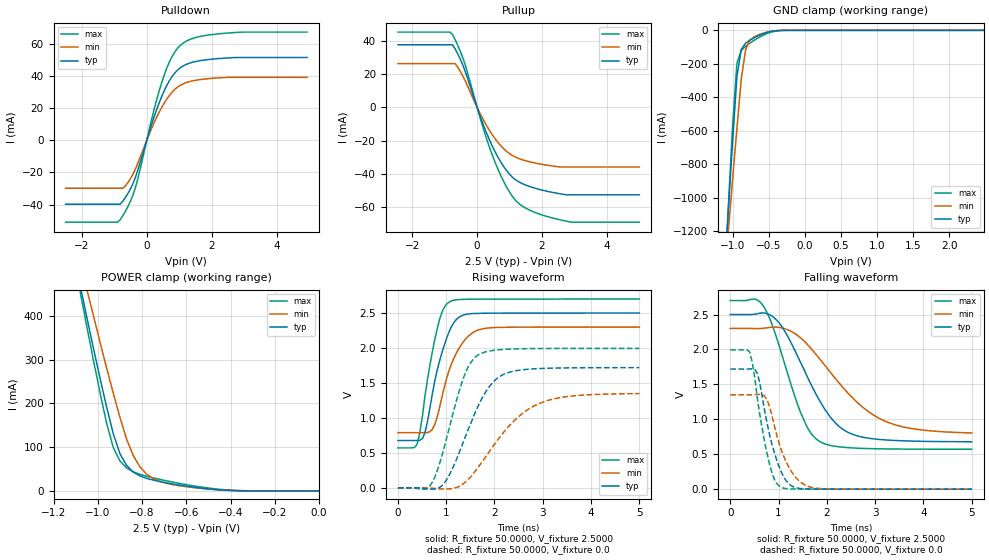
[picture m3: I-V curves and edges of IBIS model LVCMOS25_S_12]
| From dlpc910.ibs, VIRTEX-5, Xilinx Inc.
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|   Model LVCMOS25_S_12
[Model]  LVCMOS25_S_12
Model_type I/O
Polarity   Non-Inverting
Enable   Active-Low
Vinl = 0.65
Vinh = 1.85
Vmeas =  1.2500V
Cref =   0.0F
Rref =   1.0000M
Vref =   0.0V
C_comp   6.0000pF   6.0000pF   6.0000pF
[Model Spec]
Vinl   0.65   0.6   0.7
Vinh   1.85   1.7   2.0
[Temperature Range]   25.0000   85.0000   0.0
[Voltage Range]   2.5000V   2.3000V   2.7000V
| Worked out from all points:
|   slope of the pulldown table from 0 to 0.375 V, typ, clamps not added: 16.3 ohm
|   slope of the pullup table from 0 to 0.375 V, typ, clamps not added: 19.5 ohm
|   GND clamp passes 1 mA (typ) near -0.35 V on its own axis
|   POWER clamp passes 1 mA (typ) near -0.40 V on its own axis
|   rising waveform, R_fixture 50.0000, V_fixture 2.5000: 20-80 % time 370ps typ, 426ps min, 312ps max; typ from 0.677 V to 2.5 V
|   rising waveform, R_fixture 50.0000, V_fixture 0.0: 20-80 % time 648ps typ, 971ps min, 486ps max; typ from 0 V to 1.72 V
|   falling waveform, R_fixture 50.0000, V_fixture 2.5000: 20-80 % time 831ps typ, 1.19ns min, 613ps max; typ from 2.5 V to 0.679 V
|   falling waveform, R_fixture 50.0000, V_fixture 0.0: 20-80 % time 350ps typ, 399ps min, 293ps max; typ from 1.72 V to 0 V
[Pulldown]
|Voltage   I(typ)   I(min)   I(max)
-2.5V     -39.8mA    -29.84mA   -51mA
-900mV    -39.8mA    -29.84mA   -51mA
-820mV    -39.8mA    -29.84mA   -49.53mA
-660mV    -35.7mA    -28.49mA   -44.35mA
-340mV    -22.55mA   -17.45mA   -28.94mA
220mV     14.2mA     10.7mA     18.76mA
540mV     30.98mA    23.3mA     40.82mA
780mV     39.81mA    30.03mA    52.29mA
1.1V      46.18mA    35.06mA    60.36mA
1.5V      49.17mA    37.49mA    64.12mA
2.22V     51.04mA    39.01mA    66.47mA
4.94V     51.73mA    39.36mA    67.56mA
[Pullup]
|Voltage   I(typ)   I(min)   I(max)
-2.44V    37.46mA    26.15mA    45.04mA
-840mV    37.46mA    26.15mA    45.04mA
-760mV    37.46mA    26.15mA    43.62mA
-600mV    32.11mA    24.14mA    37.29mA
-360mV    21.09mA    15.58mA    24.96mA
120mV     -6.701mA   -4.795mA   -8.164mA
520mV     -25.32mA   -17.91mA   -31.29mA
920mV     -38.23mA   -26.59mA   -48.16mA
1.32V     -45.02mA   -30.95mA   -58.15mA
1.96V     -49.41mA   -34.03mA   -64.25mA
2.92V     -52.44mA   -35.78mA   -68.84mA
5V        -52.44mA   -35.78mA   -68.84mA
[GND_clamp]
|Voltage   I(typ)   I(min)   I(max)
-2.5V     -11.29A    -8.704A    -13.53A
-1.12V    -1.497A    -1.51A     -1.57A
-1.06V    -1.075A    -1.198A    -1.059A
-1V       -662mA     -888.5mA   -563.2mA
-940mV    -273.6mA   -582.9mA   -195.1mA
-880mV    -113.7mA   -290.3mA   -119.7mA
-820mV    -76.4mA    -115.2mA   -95.07mA
-760mV    -58.66mA   -58.46mA   -76.31mA
-700mV    -44.35mA   -38.35mA   -59.24mA
-520mV    -12.14mA   -10.32mA   -18.61mA
-340mV    -602.1uA   -638.4uA   -1.401mA
2.48V     19.95nA    6.298uA    40.3nA
[POWER_clamp]
|Voltage   I(typ)   I(min)   I(max)
-2.49V    3.897A     3.398A     4.279A
-1.08V    470.7mA    523.2mA    456.9mA
-1.05V    398.2mA    462.2mA    377.2mA
-1.02V    327.1mA    401.4mA    299.7mA
-960mV    191.8mA    281.1mA    154.7mA
-930mV    130.6mA    223.5mA    98.93mA
-900mV    85.26mA    168.6mA    68.69mA
-840mV    43.25mA    81.1mA     43.8mA
-780mV    28.81mA    38.65mA    33.69mA
-690mV    18.53mA    17.37mA    23.2mA
-540mV    6.864mA    6.149mA    9.448mA
0V        21.48nA    108.1nA    47.01nA
[Ramp]
| variable   typ   min   max
dV/dt_r  1.0314/0.6471n   0.8088/0.9699n   1.1964/0.4837n
dV/dt_f  1.0929/0.8300n   0.8972/1.1858n   1.2772/0.6076n
R_load = 50.0000
[Rising Waveform]
R_fixture= 50.0000
V_fixture= 2.5000
V_fixture_min= 2.3000
V_fixture_max= 2.7000
|time   V(typ)   V(min)   V(max)
0s        676.9mV    788.8mV    571.1mV
400ps     676.9mV    788.8mV    630.1mV
560ps     790.2mV    788.8mV    1.315V
710ps     1.334V     835mV      1.934V
810ps     1.674V     1.006V     2.267V
910ps     1.931V     1.293V     2.509V
1.06ns    2.233V     1.681V     2.657V
1.36ns    2.472V     2.093V     2.696V
1.72ns    2.496V     2.269V     2.698V
5ns       2.5V       2.299V     2.7V
[Rising Waveform]
R_fixture= 50.0000
V_fixture= 0.0
|time   V(typ)   V(min)   V(max)
0s        0V         672.7nV    0V
560ps     -10.74mV   -69.38uV   -17.79mV
710ps     -19.09mV   -5.424mV   76.54mV
1.01ns    118.1mV    -16.83mV   714.2mV
1.36ns    666.2mV    62.07mV    1.577V
1.67ns    1.183V     302mV      1.904V
2.12ns    1.597V     734mV      1.976V
2.88ns    1.704V     1.192V     1.992V
3.59ns    1.716V     1.312V     1.994V
5ns       1.719V     1.348V     1.994V
[Falling Waveform]
R_fixture= 50.0000
V_fixture= 2.5000
V_fixture_min= 2.3000
V_fixture_max= 2.7000
|time   V(typ)   V(min)   V(max)
0s        2.5V       2.3V       2.7V
510ps     2.504V     2.299V     2.721V
710ps     2.521V     2.305V     2.595V
1.06ns    2.335V     2.309V     1.946V
1.46ns    1.807V     2.163V     1.091V
1.82ns    1.305V     1.892V     696.7mV
2.37ns    839.8mV    1.427V     598.2mV
3.13ns    709.2mV    998.2mV    576.8mV
3.84ns    686.8mV    859mV      572.5mV
5ns       678.6mV    804.8mV    571.3mV
[Falling Waveform]
R_fixture= 50.0000
V_fixture= 0.0
|time   V(typ)   V(min)   V(max)
0s        1.719V     1.351V     1.994V
400ps     1.72V      1.351V     1.964V
560ps     1.658V     1.354V     1.303V
710ps     1.131V     1.333V     684.5mV
810ps     791.6mV    1.188V     366.8mV
910ps     530.2mV    919.4mV    147.9mV
1.06ns    240.5mV    556.4mV    25.01mV
1.36ns    20.54mV    164.9mV    2.059mV
1.72ns    2.157mV    20.39mV    989.8uV
5ns       74.73uV    162.8uV    27.75uV
